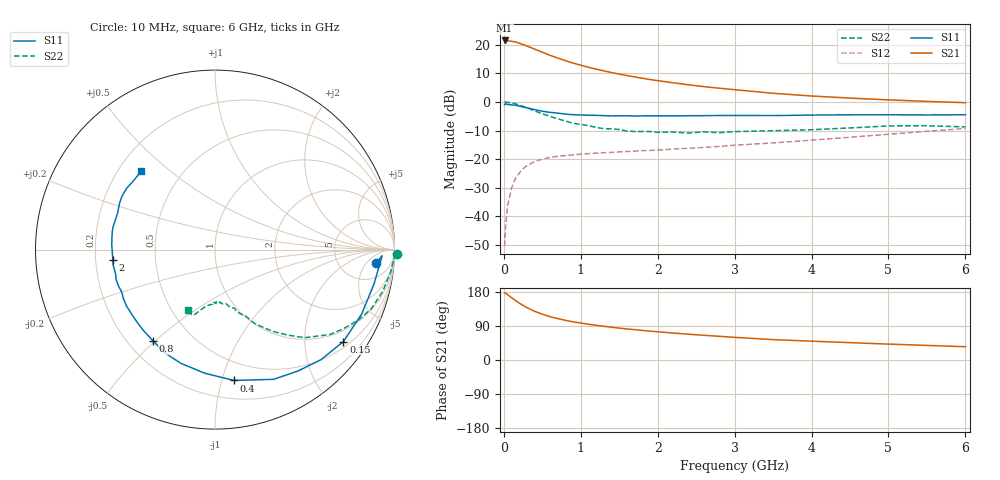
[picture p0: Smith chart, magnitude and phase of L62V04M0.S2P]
!  INFINEON TECHNOLOGIES Small Signal Semiconductors
! BFR380L3 , Si-NPN RF-Transistor in TSLP-3-1
!  Vce=2 V,  Ic=4 mA
! Common Emitter S-Parameters:  07. March 2005
#  GHz  S  MA  R  50
! f  S11  S21  S12  S22
! GHz  Mag  Ang  Mag  Ang  Mag  Ang  Mag  Ang
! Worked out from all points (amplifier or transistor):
!   36 points, 10 MHz to 6 GHz, reference 50 ohm
!   highest |S21| = 21.6 dB at 10 MHz (marker M1)
!   |S21| within 3 dB of that: start of sweep to 398.3 MHz
!   unconditionally stable (mu >= 1): 2.501 GHz to 4.73 GHz
!   at 250 MHz: K = 0.15, MSG = 21.8 dB, |S12| = -23.4 dB
!   at 1.4 GHz: K = 0.71, MSG = 14.0 dB, |S12| = -17.6 dB
!   at 6 GHz: K = 0.94, MSG = 4.5 dB, |S12| = -9.3 dB
!   S11 on the Smith chart (normalised r, x): 10 MHz: 12, -9; 150 MHz: 0.66, -2.98; 400 MHz: 0.34, -1.09; 800 MHz: 0.30, -0.49; 2 GHz: 0.27, -0.05; 6 GHz: 0.29, +0.40
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0.01  0.8993 -4.8  11.97 176.7  0.003 81.4  1.012 -1.4
0.02  0.9321 -2.1  11.91 177.2  0.0061 88.0  0.9969 -3.0
0.05  0.9064 -12.2  11.87 172.2  0.0157 86.2  0.9874 -7.1
0.1  0.8926 -23.7  11.6 164.6  0.0311 77.5  0.9628 -14.0
0.15  0.8801 -35.6  11.25 157.2  0.0458 71.6  0.9315 -20.7
0.2  0.8514 -46.1  10.72 150.1  0.0573 67.3  0.89 -26.2
0.25  0.8192 -55.7  10.16 144.2  0.0679 61.4  0.839 -31.8
0.3  0.7931 -65.7  9.559 138.2  0.0774 57.6  0.7955 -36.5
0.4  0.7365 -81.8  8.457 128.5  0.0911 50.9  0.7006 -44.5
0.5  0.6909 -94.8  7.449 120.9  0.1003 46.5  0.6238 -49.7
0.6  0.6615 -106.7  6.579 114.3  0.1074 42.9  0.5613 -54.5
0.8  0.6145 -124.2  5.305 104.7  0.1158 39.2  0.4655 -61.9
0.9  0.6013 -131.9  4.809 100.8  0.1189 38.1  0.4261 -64.1
1.1  0.5871 -142.6  4.062 94.3  0.1252 37.7  0.3856 -68.4
1.5  0.5748 -159.6  3.088 84.1  0.1339 38.6  0.3303 -75.6
2  0.572 -174.1  2.369 74.5  0.1445 42.0  0.2952 -84.0
2.2  0.5722 -178.2  2.175 71.1  0.1503 43.7  0.2979 -84.3
2.6  0.5777 174.2  1.861 65.2  0.1606 47.3  0.3008 -88.9
3.5  0.5796 159.4  1.423 53.8  0.1926 53.3  0.315 -97.8
4.5  0.5977 150.2  1.172 45.8  0.2422 59.0  0.352 -104.2
5.5  0.5945 139.7  1.026 38.5  0.3072 60.4  0.385 -110.4
6  0.5997 133.2  0.975 35.1  0.3443 59.5  0.3669 -113.9
